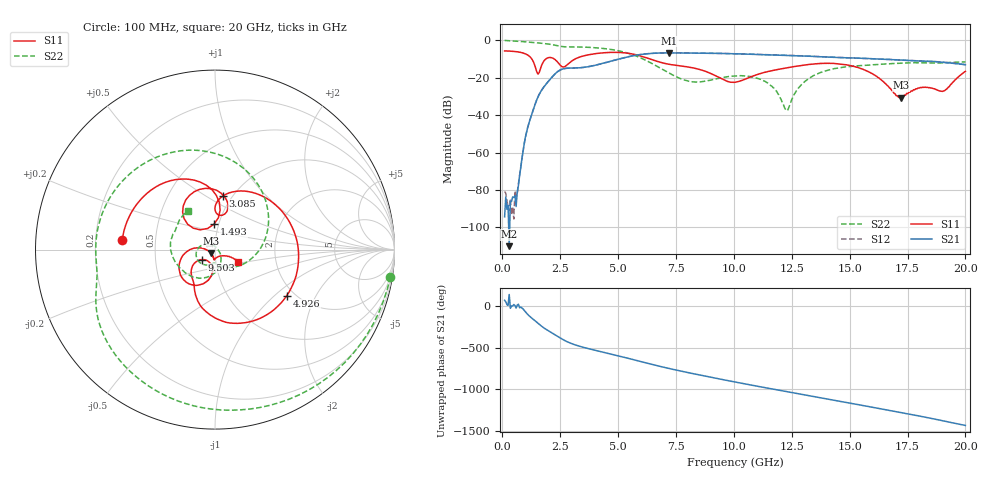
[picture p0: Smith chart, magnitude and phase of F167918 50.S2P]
!  2-Port S-parameters saved by WinCal
! VAR MeasName=S-Parameters (CALIBRATED_DATA) read from VNA (N5242A)
! VAR MeasDate=2016-11-22 10:27:15
! VAR NAME=F167918 50
! VAR FILENAME=F167918 50.S2P
! VAR DATE=2016-11-22 10:27:15
! VAR PHYS_PORTS=1,2
# Hz S DB R 50
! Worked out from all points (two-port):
!   401 points, 100 MHz to 20 GHz, reference 50 ohm
!   highest |S21| = -6.73 dB at 7.214 GHz (marker M1); lowest = -110.0 dB at 299 MHz (marker M2)
!   |S21| within 3 dB of the highest: 5.122 GHz to 15.73 GHz (10.61 GHz wide, 102 % of centre)
!   lowest |S11| = -30.7 dB at 17.21 GHz (marker M3), VSWR 1.06, Z = 47.9 - j1.9 ohm
!   |S11| at or under -10 dB: 1.273 GHz to 1.879 GHz (605.9 MHz wide, 38.4 % of centre); 2.242 GHz to 3.145 GHz (902.8 MHz wide, 33.5 % of centre); 6.378 GHz to end of sweep
!   |S22| runs from -37.7 to -0.1 dB; largest |S21 - S12| = 0.0042
!   S11 on the Smith chart (normalised r, x): 100 MHz: 0.32, +0.05; 1.493 GHz: 0.95, +0.27; 3.085 GHz: 0.91, +0.60; 4.926 GHz: 1.82, -1.20; 9.503 GHz: 0.86, -0.10; 20 GHz: 1.28, -0.18
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1e8  -5.69 174.1  -94.36 70.9  -80.78 87.3  -0.10 -8.8
2.99e8  -5.77 162.2  -110.03 139.7  -91.00 -122.7  -0.23 -25.1
6.4725e8  -6.16 140.5  -80.69 13.9  -82.29 59.0  -0.49 -52.4
1.04525e9  -7.52 111.0  -49.21 -83.4  -49.22 -82.9  -0.88 -81.1
1.493e9  -16.98 92.2  -31.66 165.5  -31.66 165.8  -1.35 -110.1
2.33875e9  -10.99 76.6  -17.29 5.1  -17.28 5.1  -2.81 -156.6
3.085e9  -10.41 81.6  -14.85 -100.5  -14.85 -100.6  -3.55 176.6
3.43325e9  -8.60 60.7  -14.60 -130.7  -14.59 -130.7  -3.61 162.1
4.92575e9  -6.46 -32.7  -10.37 127.7  -10.36 127.8  -5.38 90.8
6.7665e9  -11.56 -114.9  -6.82 -2.0  -6.81 -2.0  -14.51 -22.4
7.21425e9  -12.87 -120.9  -6.73 -31.2  -6.71 -31.1  -17.65 -49.2
8.259e9  -14.79 -136.9  -6.83 -94.0  -6.81 -93.9  -22.29 -90.9
9.50275e9  -20.71 -143.0  -7.05 -163.4  -7.05 -163.5  -19.96 -121.4
1.005e10  -22.44 -118.0  -7.20 167.0  -7.21 167.0  -19.07 -141.4
1.1443e10  -16.81 -98.0  -7.75 93.8  -7.69 93.9  -22.66 158.9
1.228875e10  -14.76 -104.3  -8.05 50.2  -8.02 50.2  -37.65 38.4
1.338325e10  -12.77 -120.4  -8.59 -5.8  -8.54 -5.8  -19.32 -80.5
1.5025e10  -13.51 -159.1  -9.45 -88.2  -9.40 -88.5  -13.99 -132.4
1.67165e10  -25.35 176.6  -10.23 -175.2  -10.29 -175.1  -12.56 -166.8
1.7214e10  -30.67 -137.3  -10.57 158.9  -10.56 158.7  -12.25 -176.7
1.905475e10  -27.09 -57.3  -11.74 58.4  -11.72 58.2  -12.08 147.7
2e10  -16.62 -28.1  -13.07 3.7  -13.01 3.9  -11.60 125.4
